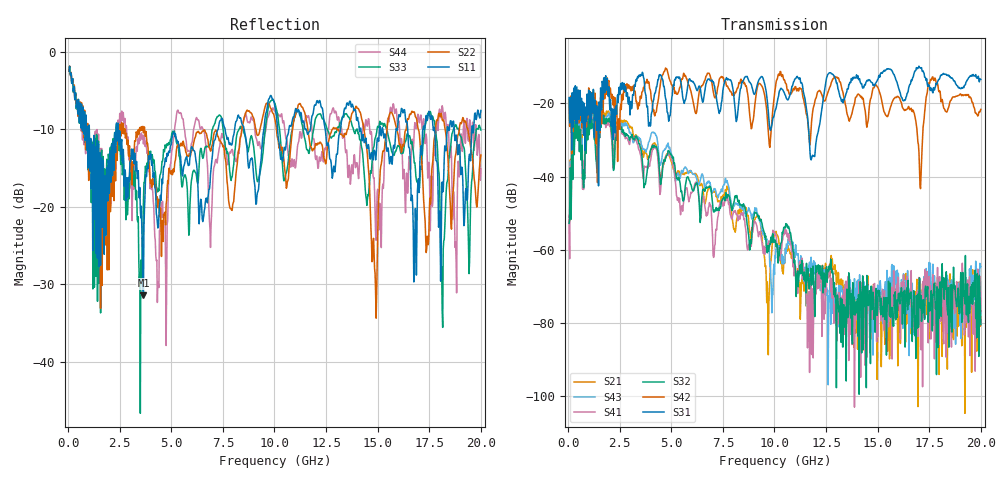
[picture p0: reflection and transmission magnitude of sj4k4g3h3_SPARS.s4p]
! FILE: E:\users\goganessyan\GBX_Backplane\FR408_backplane\1m_OUTBOUND_FEXT\sj4k4g3h3_SPARS.s4p
# MHZ S RI R 50.00
! FREQ  S11  S12  S13  S14
!  S21  S22  S23  S24
!  S31  S32  S33  S34
!  S41  S42  S43  S44
!  REAL  IMAG  REAL  IMAG  REAL  IMAG  REAL  IMAG
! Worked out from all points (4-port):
!   799 points, 50 MHz to 20 GHz, reference 50 ohm
!   strongest paths, dB at 50 MHz, 5.025 GHz, 10.03 GHz, 15.03 GHz, 20 GHz:
!     S31: -18.4, -18.5, -22.1, -13.3, -13.5
!     S42: -19.2, -15.0, -16.3, -15.8, -21.6
!     S32: -52.8, -34.2, -57.3, -71.1, -80.4
!     S41: -50.5, -35.7, -55.9, -73.7, -76.9
!     S43: -51.0, -34.1, -61.6, -72.7, -64.6
!     S21: -52.4, -36.2, -55.6, -75.0, -78.4
!   lowest |S11| = -31.4 dB at 3.65 GHz (marker M1), VSWR 1.06, Z = 52.6 - j0.952 ohm
!   |S11| at or under -10 dB: 1.027 GHz to 2.329 GHz (1.302 GHz wide, 77.6 % of centre); 2.437 GHz to 7.269 GHz (4.832 GHz wide, 99.6 % of centre); 8.529 GHz to 9.485 GHz (956.1 MHz wide, 10.6 % of centre)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
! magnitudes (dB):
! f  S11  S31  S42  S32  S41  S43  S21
! 50 MHz  -2.5  -18.4  -19.2  -52.8  -50.5  -51.0  -52.4
! 425 MHz  -6.3  -15.5  -16.4  -24.7  -25.4  -23.5  -22.9
! 3.65 GHz  -31.4  -12.8  -15.7  -39.7  -40.6  -32.4  -34.7
! 9.9 GHz  -6.1  -24.9  -23.0  -56.1  -56.0  -72.6  -57.7
! 14.9 GHz  -14.0  -14.5  -14.9  -74.2  -78.6  -82.0  -79.8
! 18.12 GHz  -16.8  -12.1  -18.9  -63.8  -74.4  -69.0  -89.1
! 20 GHz  -7.6  -13.5  -21.6  -80.4  -76.9  -64.6  -78.4
